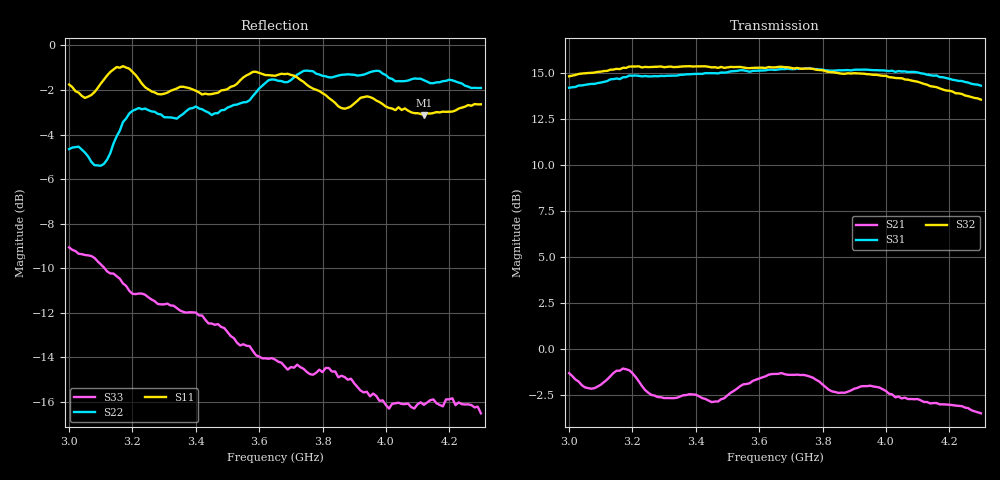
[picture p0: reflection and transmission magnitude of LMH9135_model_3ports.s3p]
! Created Sun May  3 23:42:57 2020
# hz S ri R 50
! 3 Port Network Data from SP1.SP block
! freq  reS11  imS11  reS12  imS12  reS13  imS13
!  reS21  imS21
!  reS22  imS22  reS23  imS23
!  reS31  imS31  reS32  imS32
!  reS33  imS33
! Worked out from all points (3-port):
!   131 points, 3 GHz to 4.3 GHz, reference 50 ohm
!   strongest paths, dB at 3 GHz, 3.32 GHz, 3.65 GHz, 3.98 GHz, 4.3 GHz:
!     S32: 14.8, 15.3, 15.3, 14.9, 13.5
!     S31: 14.2, 14.8, 15.1, 15.1, 14.3
!     S21: -1.3, -2.7, -1.3, -2.1, -3.5
!   lowest |S11| = -3.1 dB at 4.12 GHz (marker M1), VSWR 5.63, Z = 147 + j136 ohm
!   |S11| at or under -10 dB: nowhere
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3e9  -0.8159 -0.0445  0.3522 -0.2078  -0.0385 0.0726
     -0.8435 0.1726  0.393 -0.4335  -0.0526 0.0591
     4.738 1.932  -5.143 -1.931  -0.2827 -0.2101
3.17e9  -0.859 0.2626  0.3687 -0.3964  -0.0388 0.0667
        -0.7301 0.5031  0.2337 -0.631  -0.0563 0.063
        5.428 -0.6003  -5.747 0.7339  -0.2869 -0.0565
3.29e9  -0.6569 0.4141  0.1756 -0.5305  -0.0261 0.0657
        -0.441 0.5954  -0.0511 -0.698  -0.0426 0.067
        4.945 -2.428  -5.2 2.664  -0.2582 0.0472
3.46e9  -0.4908 0.6069  -0.0218 -0.5954  -0.0258 0.0627
        -0.2129 0.6891  -0.3081 -0.6331  -0.0391 0.0695
        3.421 -4.438  -3.469 4.668  -0.1934 0.1355
3.65e9  -0.1345 0.844  -0.2999 -0.6692  -0.0361 0.078
        0.1298 0.8472  -0.5416 -0.6388  -0.0439 0.0908
        0.8551 -5.653  -0.8734 5.743  -0.0732 0.1834
3.76e9  0.1642 0.7901  -0.5379 -0.5651  -0.0272 0.0912
        0.3975 0.7435  -0.7384 -0.4718  -0.0287 0.104
        -0.8801 -5.717  0.8756 5.699  -0.0117 0.1827
3.91e9  0.4063 0.6315  -0.7177 -0.3311  -0.0204 0.0941
        0.5387 0.5713  -0.8197 -0.2452  -0.0207 0.1054
        -2.978 -4.891  2.864 4.808  0.0537 0.1627
4e9  0.5555 0.4723  -0.8218 -0.1439  -0.0134 0.1053
     0.6391 0.4307  -0.8547 -0.0748  -0.00949 0.1154
     -3.648 -4.37  3.533 4.23  0.0868 0.1297
4.12e9  0.6565 0.2378  -0.8495 0.1243  -0.00392 0.1124
        0.6725 0.2552  -0.8233 0.1409  0.0032 0.1204
        -5.048 -2.386  4.72 2.28  0.1357 0.0773
4.3e9  0.7125 -0.1904  -0.7654 0.5749  0.0213 0.1319
       0.6694 -0.0334  -0.6836 0.4205  0.0302 0.1359
       -5.178 0.2309  4.748 -0.1616  0.1489 0.0137
